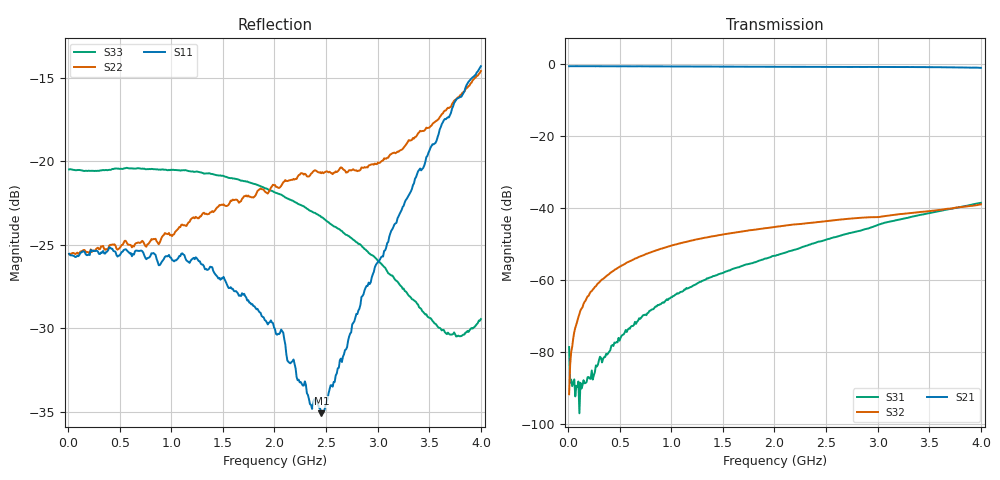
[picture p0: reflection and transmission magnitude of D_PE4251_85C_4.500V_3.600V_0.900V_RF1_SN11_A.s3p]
! Device ID: PE4251_SoldCshunt_081809
! Dir: c:\Test Bench Repositories\Bench_Software_CVI_Version_8\trunk\PSC 4Port_VNA Bench\datalog\4250\TEST\PE4251_SoldCshunt_081809\85C\4p500000\RF1
! Serial: 11
! Insertion: A
! Temp: 85C
! VDD: 4.500
! Control_Hi: 80.000
! Control_Lo: 20.000
! Logic State: RF1
! Port 1: RFC
! Port 2: RF1
! Port 3: RF2
! V1 = 0.90
! V2 = 3.60
! V3 = 0.90
! IDD: 5.897570e-05
! FILE NAME
! DATE 08/18/09  20:18
! CORRECTED  DATA
#  Hz  S  RI  R  50.00
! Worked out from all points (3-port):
!   401 points, 10 MHz to 4 GHz, reference 50 ohm
!   strongest paths, dB at 10 MHz, 1.008 GHz, 2.005 GHz, 3.002 GHz, 4 GHz:
!     S21: -0.6, -0.7, -0.8, -0.8, -1.1
!     S32: -91.9, -50.4, -45.3, -42.6, -39.0
!     S31: -78.7, -64.9, -53.3, -44.7, -38.6
!   lowest |S11| = -35.1 dB at 2.454 GHz (marker M1), VSWR 1.04, Z = 49.9 - j1.76 ohm
!   |S11| at or under -10 dB: start of sweep to end of sweep
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1e7  0.0528 2.05e-05  0.931 -0.00418  -2.51e-05 -1.75e-08
     0.9305 -0.00507  0.0528 9.74e-05  8.65e-05 -5.2e-05
     0.000111 -3.32e-05  1.31e-05 -2.19e-05  0.0946 -0.000221
1.696e8  0.0528 7.39e-08  0.9298 -0.0587  2.94e-06 -3.79e-05
         0.9294 -0.0581  0.0537 8.85e-05  5.49e-05 0.000517
         1.45e-05 -3.36e-05  5.83e-05 0.00051  0.0937 -0.00362
3.79075e8  0.0535 -0.00439  0.9212 -0.1273  -5.51e-05 -7.43e-05
           0.921 -0.1269  0.0543 -0.00351  0.000102 0.00116
           -5.86e-05 -6.98e-05  0.000101 0.00114  0.0936 -0.00976
4.98775e8  0.0519 -0.00616  0.9131 -0.1671  -0.000127 -8.27e-05
           0.9134 -0.1663  0.0547 -0.00505  0.000149 0.00151
           -0.000111 -8.85e-05  0.000161 0.00151  0.0941 -0.0124
7.0825e8  0.0533 -0.009  0.8989 -0.2338  -0.000285 -9.52e-05
          0.8982 -0.2339  0.0565 -0.00987  0.000244 0.00212
          -0.000283 -9.06e-05  0.000247 0.00212  0.0937 -0.0161
1.14715e9  0.0473 -0.0177  0.8475 -0.3679  -0.000753 -7.26e-05
           0.8481 -0.3675  0.061 -0.0197  0.000547 0.00331
           -0.000763 -9.1e-05  0.000559 0.00332  0.0909 -0.0238
2.005e9  0.0258 -0.0178  0.7024 -0.5833  -0.00218 0.000155
         0.702 -0.5833  0.0716 -0.0456  0.00099 0.00532
         -0.00215 0.000142  0.000965 0.00533  0.0747 -0.0305
2.453875e9  -0.000315 -0.0176  0.6095 -0.6743  -0.00342 0.000236
            0.6083 -0.6748  0.0615 -0.0686  0.00105 0.0063
            -0.00342 0.000242  0.00103 0.00633  0.0602 -0.0317
3.670825e9  -0.1132 -0.0733  0.2739 -0.8575  -0.009 0.00287
            0.2762 -0.8562  -0.0644 -0.1285  -0.000123 0.00965
            -0.00903 0.00282  -0.000162 0.00968  0.00411 -0.0301
4e9  -0.1761 -0.0786  0.1561 -0.8726  -0.0109 0.00437
     0.1556 -0.8703  -0.1369 -0.1267  -0.000754 0.0111
     -0.0109 0.00437  -0.000786 0.0111  -0.0155 -0.0299
